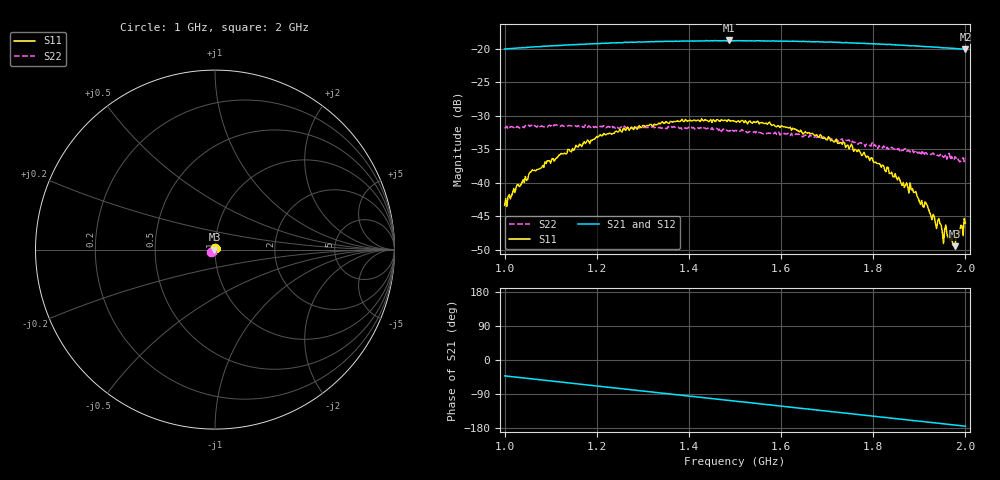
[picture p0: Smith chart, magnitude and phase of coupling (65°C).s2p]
!Agilent Technologies,E8363C,MY43030407,A.09.42.15
!Agilent E8363C: A.09.42.15
!Date: Friday, September 05, 2025 17:51:10
!Correction: S11(Full 2 Port(1,2))
!S21(Full 2 Port(1,2))
!S12(Full 2 Port(1,2))
!S22(Full 2 Port(1,2))
!S2P File: Measurements: S11, S21, S12, S22:
# Hz S  dB  R 50
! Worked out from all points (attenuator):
!   401 points, 1 GHz to 2 GHz, reference 50 ohm
!   highest |S21| = -18.78 dB at 1.488 GHz (marker M1); lowest = -20.1 dB at 2 GHz (marker M2)
!   lowest |S11| = -49.5 dB at 1.978 GHz (marker M3), VSWR 1.01, Z = 49.7 - j0.0844 ohm
!   |S11| at or under -10 dB: start of sweep to end of sweep
!   |S22| runs from -36.9 to -31.4 dB; largest |S21 - S12| = 0.0012
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1e9  -43.42 76.9  -20.05 -41.9  -20.05 -42.0  -31.91 -142.1
1.0575e9  -38.38 74.0  -19.77 -49.6  -19.79 -49.6  -31.43 -144.4
1.1675e9  -34.63 56.3  -19.36 -64.3  -19.36 -64.2  -31.56 -147.0
1.2625e9  -32.22 41.3  -19.05 -76.9  -19.10 -77.0  -31.80 -151.4
1.335e9  -31.12 31.4  -18.93 -86.5  -18.95 -86.5  -31.82 -153.7
1.4875e9  -30.68 6.0  -18.78 -106.7  -18.81 -106.7  -32.29 -156.3
1.5e9  -30.83 5.9  -18.83 -108.3  -18.83 -108.2  -32.24 -156.1
1.5725e9  -31.12 -7.5  -18.85 -118.1  -18.86 -118.0  -32.59 -158.4
1.6675e9  -32.64 -26.5  -19.00 -130.5  -18.98 -130.6  -33.14 -160.3
1.75e9  -34.60 -43.8  -19.14 -141.6  -19.15 -141.5  -33.88 -159.7
1.835e9  -38.65 -62.1  -19.36 -152.9  -19.40 -152.8  -34.79 -160.4
1.885e9  -40.89 -84.0  -19.57 -159.6  -19.57 -159.3  -35.09 -159.6
1.905e9  -42.66 -91.2  -19.65 -162.0  -19.65 -162.1  -35.44 -159.5
1.9175e9  -43.48 -99.7  -19.71 -163.9  -19.72 -163.6  -35.77 -161.0
1.9325e9  -45.08 -105.0  -19.78 -165.7  -19.76 -165.7  -35.81 -158.4
1.945e9  -46.16 -119.6  -19.83 -167.5  -19.84 -167.4  -35.88 -157.6
1.95e9  -47.44 -118.9  -19.87 -168.0  -19.83 -168.0  -36.03 -158.5
1.96e9  -47.68 -135.7  -19.90 -169.4  -19.91 -169.2  -36.50 -155.6
1.9725e9  -49.31 -165.5  -19.95 -171.1  -19.97 -171.0  -36.48 -157.0
1.9775e9  -49.49 -165.3  -19.98 -171.7  -19.99 -171.6  -36.14 -157.8
1.9875e9  -47.66 170.2  -20.02 -173.0  -20.07 -173.1  -36.89 -155.6
2e9  -46.07 158.0  -20.11 -174.7  -20.12 -174.6  -36.35 -154.4
